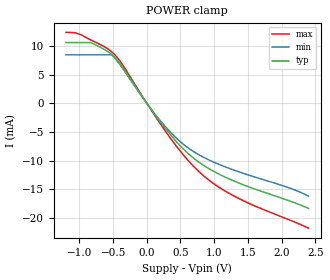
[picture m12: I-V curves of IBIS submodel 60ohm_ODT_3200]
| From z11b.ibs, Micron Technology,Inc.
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| SUBMODEL 60ohm_ODT_3200
[Submodel]   60ohm_ODT_3200
Submodel_type  Dynamic_clamp
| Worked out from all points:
|   POWER clamp passes 1 mA (typ) near -0.06 V on its own axis
[POWER Clamp]
|   Voltage   I(typ)   I(min)   I(max)
-1.2V     10.59mA    8.445mA    12.36mA
-1.045V   10.59mA    8.445mA    12.22mA
-830mV    10.59mA    8.445mA    11.02mA
-515mV    8.434mA    8.341mA    8.897mA
-370mV    6.438mA    6.267mA    6.886mA
0V        51.68nA    48.39nA    53.27nA
310mV     -4.9mA     -4.531mA   -5.424mA
570mV     -8.284mA   -7.406mA   -9.394mA
855mV     -10.92mA   -9.496mA   -12.77mA
1.15V     -12.8mA    -11.03mA   -15.22mA
1.43V     -14.2mA    -12.21mA   -16.98mA
2.4V      -18.34mA   -16.19mA   -21.77mA
